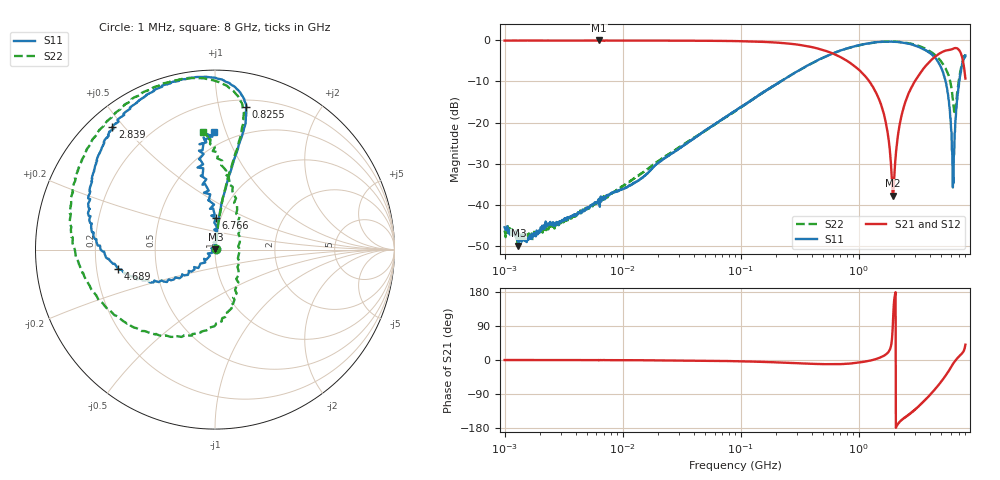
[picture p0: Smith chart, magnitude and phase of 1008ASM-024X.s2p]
!s-Parameter Generated by FASTRON Sdn. Bhd.
!FASTRON P/N : 1008ASM-024X
!Keysight Technologies: E5071C_MY46733604_B.14.02
!Date: Wed Jun 19 15:45:22 2024
!Version  :Rev00  Wed Jun 19 15:45:22 2024
!Data & Calibration Information:
!Freq  S11:SOLT2(ON)  S21:SOLT2(ON)  S12:SOLT2(ON)  S22:SOLT2(ON)
!PortZ  Port1:50+j0  Port2:50+j0
!When reading reference impedance value at option line is always used.
! Remarks : This data is being provided solely for informational purposes.
# Hz S dB R 50
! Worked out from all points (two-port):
!   1601 points, 1 MHz to 8 GHz, reference 50 ohm
!   highest |S21| = -0.01 dB at 6.301 MHz (marker M1); lowest = -37.8 dB at 1.955 GHz (marker M2)
!   |S21| within 3 dB of the highest: start of sweep to 581.9 MHz; 4.939 GHz to 7.292 GHz (2.353 GHz wide, 38.5 % of centre)
!   lowest |S11| = -50.0 dB at 1.31 MHz (marker M3), VSWR 1.01, Z = 50.3 + j0.172 ohm
!   |S11| at or under -10 dB: start of sweep to 217.9 MHz; 5.434 GHz to 7.095 GHz (1.661 GHz wide, 26.5 % of centre)
!   |S22| runs from -50.1 to -0.3 dB; largest |S21 - S12| = 0.0087
!   S11 on the Smith chart (normalised r, x): 1 MHz: 1.01, +0.00; 825.5 MHz: 0.26, +1.21; 2.839 GHz: 0.07, +0.46; 4.689 GHz: 0.29, -0.09; 6.766 GHz: 0.95, +0.34; 8 GHz: 0.39, +0.91
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1000000  -45.50 21.1  -0.04 -0.1  -0.03 -0.2  -46.30 13.8
1310238  -50.00 32.7  -0.04 -0.1  -0.03 -0.1  -47.00 5.2
4479405  -41.70 62.5  -0.04 -0.2  -0.03 -0.2  -41.70 66.0
6301378  -39.30 53.7  -0.01 -0.5  -0.02 -0.4  -39.30 74.7
2.00676e7  -29.80 80.5  -0.05 -0.8  -0.05 -0.7  -29.40 80.0
8.994653e7  -17.10 83.7  -0.17 -3.2  -0.16 -3.1  -17.20 83.0
4.006501e8  -5.57 77.8  -1.63 -10.0  -1.63 -10.0  -5.60 78.3
8.255136e8  -1.81 77.6  -5.27 -9.7  -5.27 -9.6  -1.84 79.0
1.395953e9  -0.44 88.3  -12.70 2.5  -12.70 2.6  -0.48 91.5
1.645766e9  -0.32 94.2  -18.40 11.8  -18.40 11.9  -0.31 98.7
1.7949e9  -0.29 98.4  -24.40 22.5  -24.40 22.5  -0.27 104.0
1.954687e9  -0.35 103.0  -37.80 113.0  -37.80 113.0  -0.31 109.0
2.222796e9  -0.43 111.0  -20.40 -163.0  -20.40 -163.0  -0.36 119.0
2.839031e9  -1.01 130.0  -11.10 -137.0  -11.10 -137.0  -0.86 142.0
3.710194e9  -2.50 158.0  -6.15 -103.0  -6.16 -103.0  -2.15 -180.0
4.688537e9  -5.16 -169.0  -3.43 -67.7  -3.44 -67.7  -4.22 -134.0
5.584277e9  -11.50 -144.0  -2.40 -36.1  -2.41 -36.0  -7.58 -89.4
6.226476e9  -32.00 -132.0  -2.08 -12.1  -2.09 -12.0  -13.90 -54.2
6.457806e9  -24.80 81.0  -1.89 -4.9  -1.91 -4.8  -17.40 -12.4
6.766244e9  -15.10 88.4  -1.91 3.0  -1.92 3.2  -13.80 50.8
7.306013e9  -7.54 101.0  -3.07 14.1  -3.06 14.3  -7.05 81.9
8e9  -3.65 90.6  -9.29 40.4  -9.26 40.6  -3.64 95.6
